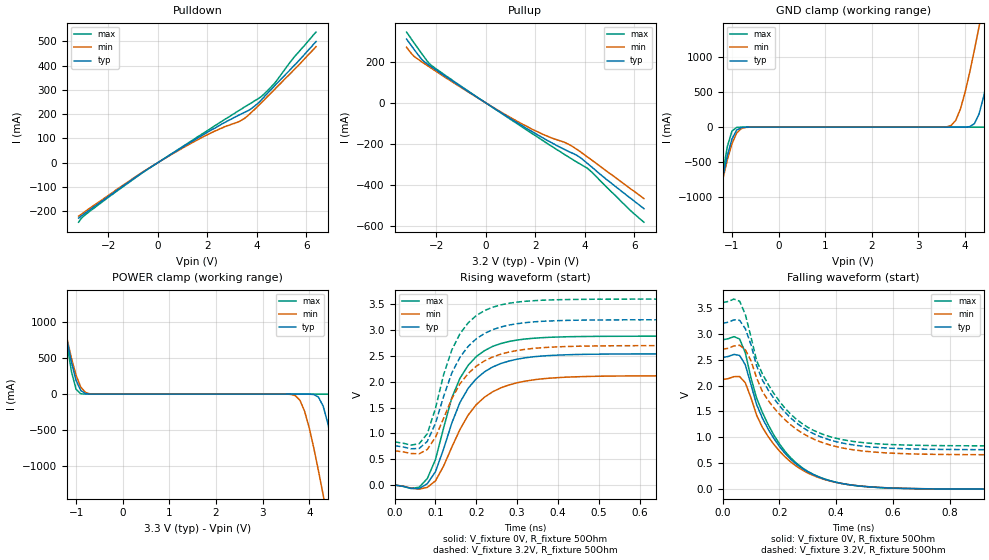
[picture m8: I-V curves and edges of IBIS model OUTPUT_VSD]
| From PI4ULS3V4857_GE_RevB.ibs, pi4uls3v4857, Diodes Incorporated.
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[Model]  OUTPUT_VSD
Model_type  Output
Vmeas=1.6
|Variable   typ   min   max
C_comp   7.59p   7.49p   7.74p
|Variable   typ   min   max
[Voltage Range]   3.2   2.7   3.6
[Temperature Range]   40   85   -40
[Pullup Reference]   3.2   2.7   3.6
[Pulldown Reference]   0   0   0
[Power Clamp Reference]   3.3   2.9   3.6
[GND Clamp Reference]   0   0   0
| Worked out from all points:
|   slope of the pulldown table from 0 to 0.48 V, typ, clamps not added: 15.6 ohm
|   slope of the pullup table from 0 to 0.48 V, typ, clamps not added: 13 ohm
|   GND clamp passes 1 mA (typ) near -0.71 V on its own axis
|   POWER clamp passes 1 mA (typ) near -0.71 V on its own axis
|   falling waveform, V_fixture 0V, R_fixture 50Ohm: 20-80 % time 155ps typ, 161ps min, 152ps max; typ from 2.54 V to 0 V
|   falling waveform, V_fixture 3.2V, R_fixture 50Ohm: 20-80 % time 164ps typ, 173ps min, 157ps max; typ from 3.2 V to 0.761 V
|   rising waveform, V_fixture 0V, R_fixture 50Ohm: 20-80 % time 85.9ps typ, 96.1ps min, 76.5ps max; typ from 0 V to 2.54 V
|   rising waveform, V_fixture 3.2V, R_fixture 50Ohm: 20-80 % time 81.9ps typ, 91ps min, 75.3ps max; typ from 0.761 V to 3.2 V
[GND Clamp]
-3.3V     -9.7A      -8.62A     -12.6A
-1.4V     -1.47A     -1.4A      -1.65A
-1.1V     -409mA     -469mA     -279mA
-900mV    -43.4mA    -85.5mA    -4.58mA
3.7V      9.32nA     23.4mA     22.8pA
3.9V      13.9uA     259mA      25.2pA
4.2V      49.7mA     1.1A       4.57nA
4.3V      189mA      1.43A      630nA
4.5V      761mA      2.12A      4.66mA
4.7V      1.5A       2.84A      311mA
5V        2.73A      3.95A      1.75A
6.6V      9.7A       10.1A      11.2A
[POWER Clamp]
-3.3V     9.7A       8.51A      13.1A
-1.4V     1.5A       1.43A      1.75A
-1.1V     440mA      496mA      311mA
-900mV    49.7mA     97mA       4.66mA
3.7V      -13.9nA    -20.8mA    -22.8pA
3.9V      -19.2uA    -237mA     -25.2pA
4.2V      -43.4mA    -1.07A     -6.82nA
4.3V      -170mA     -1.4A      -910nA
4.5V      -725mA     -2.11A     -4.58mA
4.7V      -1.47A     -2.84A     -279mA
5V        -2.69A     -3.97A     -1.65A
6.6V      -9.7A      -10.2A     -10.8A
[Pulldown]
| Voltage   I(typ)   I(min)  I(max)
-3.2V     -228mA     -220mA     -245mA
-3V       -213mA     -206mA     -220mA
-2.1V     -147mA     -142mA     -150mA
-600mV    -39.2mA    -37.6mA    -40.2mA
500mV     32.1mA     30.6mA     33.2mA
1.8V      113mA      105mA      119mA
3.5V      207mA      182mA      229mA
4V        240mA      228mA      260mA
4.3V      271mA      258mA      283mA
4.7V      314mA      299mA      324mA
5.5V      399mA      382mA      433mA
6.4V      499mA      478mA      538mA
[Pullup]   |Note: Vtable = Vcc - Voutput
| Voltage   I(typ)   I(min)  I(max)
-3.2V     311mA      271mA      345mA
-2.9V     261mA      227mA      293mA
-2.6V     214mA      201mA      242mA
-2.2V     176mA      169mA      183mA
-700mV    54.9mA     52.3mA     56.8mA
1V        -76.5mA    -71.4mA    -80.1mA
2.3V      -170mA     -153mA     -183mA
3.4V      -240mA     -205mA     -268mA
3.7V      -257mA     -228mA     -290mA
4.1V      -294mA     -263mA     -318mA
5.8V      -460mA     -414mA     -519mA
6.4V      -516mA     -467mA     -582mA
[Falling Waveform]
V_fixture = 0V
V_fixture_min = 0V
V_fixture_max = 0V
R_fixture = 50Ohm
C_fixture = 0F
|   Time   V(typ)   V(min)   V(max)
0s        2.54V      2.116V     2.882V
60ps      2.581V     2.173V     2.898V
80ps      2.4V       2.053V     2.632V
120ps     1.629V     1.424V     1.755V
160ps     1.164V     1.019V     1.251V
220ps     690.7mV    623.8mV    728.5mV
300ps     334.4mV    312.5mV    343.6mV
380ps     160.2mV    154.4mV    160.3mV
660ps     12.26mV    13.43mV    11.28mV
1.98ns    65.51uV    72.94uV    41.98uV
[Falling Waveform]
V_fixture = 3.2V
V_fixture_min = 2.7V
V_fixture_max = 3.6V
R_fixture = 50Ohm
C_fixture = 0F
|   Time   V(typ)   V(min)   V(max)
0s        3.2V       2.7V       3.6V
60ps      3.258V     2.778V     3.628V
80ps      3.098V     2.692V     3.374V
120ps     2.377V     2.145V     2.479V
140ps     2.109V     1.887V     2.227V
200ps     1.612V     1.449V     1.697V
280ps     1.198V     1.084V     1.266V
380ps     946.6mV    850.1mV    1.01V
660ps     777.4mV    681.8mV    849.6mV
1.98ns    760.6mV    662.4mV    834.8mV
[Rising Waveform]
V_fixture = 0V
V_fixture_min = 0V
V_fixture_max = 0V
R_fixture = 50Ohm
C_fixture = 0F
|   Time   V(typ)   V(min)   V(max)
0s        0V         0V         0V
60ps      -67.72mV   -79.82mV   -42.62mV
80ps      27mV       -44.65mV   127.1mV
100ps     259.3mV    81.53mV    495.9mV
140ps     1.201V     733.6mV    1.689V
160ps     1.599V     1.076V     2.067V
200ps     2.059V     1.557V     2.487V
280ps     2.4V       1.937V     2.779V
500ps     2.533V     2.106V     2.878V
1.98ns    2.54V      2.116V     2.882V
[Rising Waveform]
V_fixture = 3.2V
V_fixture_min = 2.7V
V_fixture_max = 3.6V
R_fixture = 50Ohm
C_fixture = 0F
|   Time   V(typ)   V(min)   V(max)
0s        760.6mV    662.3mV    834.7mV
60ps      708.2mV    604.9mV    799.8mV
80ps      845.1mV    689mV      994.4mV
100ps     1.198V     926.2mV    1.487V
120ps     1.717V     1.294V     2.139V
160ps     2.474V     1.961V     2.929V
200ps     2.831V     2.301V     3.281V
280ps     3.097V     2.574V     3.519V
520ps     3.196V     2.695V     3.597V
1.98ns    3.2V       2.7V       3.6V
[Ramp]
|   typ   min   max
dV/dt_r   2.09/5.54E-11   1.76/6.34E-11   2.36/4.99E-11
dV/dt_f   2.09/1.58E-10   1.75/1.65E-10   2.36/1.55E-10
R_load =   50.0000
